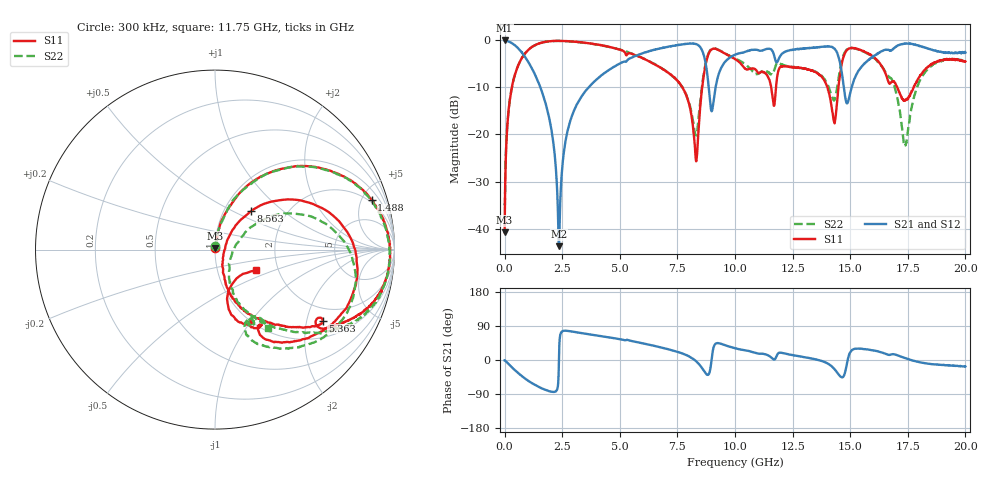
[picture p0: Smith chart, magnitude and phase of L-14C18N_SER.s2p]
!P/N: L-14C18NJV4
!Agilent N5230A: A.07.50.26
!Date: Tuesday, October 28, 2008 10:37:53
!Correction: S11(Full 2 Port(1,2))
!S21(Full 2 Port(1,2))
!S12(Full 2 Port(1,2))
!S22(Full 2 Port(1,2))
!S2P File: Measurements: S11, S21, S12, S22:
# Hz S  dB  R 50
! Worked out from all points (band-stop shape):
!   1601 points, 300 kHz to 20 GHz, reference 50 ohm
!   highest |S21| = -0.12 dB at 300 kHz (marker M1); lowest = -43.7 dB at 2.363 GHz (marker M2)
!   |S21| within 3 dB of the highest: 5.822 GHz to 8.64 GHz (2.817 GHz wide, 39 % of centre); 16.13 GHz to end of sweep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
!   lowest |S11| = -40.8 dB at 300 kHz (marker M3), VSWR 1.02, Z = 49.9 + j0.912 ohm
!   |S11| at or under -10 dB: 7.709 GHz to 8.575 GHz (865.7 MHz wide, 10.6 % of centre); 14 GHz to 14.49 GHz (487.4 MHz wide, 3.42 % of centre); 17.04 GHz to 17.76 GHz (714.2 MHz wide, 4.11 % of centre)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
!   |S22| runs from -34.9 to -0.2 dB; largest |S21 - S12| = 0.022
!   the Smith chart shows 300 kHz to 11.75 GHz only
!   S11 on the Smith chart (normalised r, x): 300 kHz: 1.00, +0.02; 1.488 GHz: 1.76, +5.98; 5.363 GHz: 1.53, -2.49; 8.563 GHz: 1.34, +0.63; 11.75 GHz: 1.54, -0.38
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300000  -40.76 94.4  -0.12 -0.9  -0.14 -0.5  -34.64 96.2
3.627946e8  -8.93 65.7  -0.85 -22.1  -0.85 -22.1  -8.96 65.5
1.487778e9  -0.77 17.5  -9.23 -71.4  -9.24 -71.4  -0.78 17.2
2.037769e9  -0.26 3.3  -19.18 -83.7  -19.20 -83.9  -0.27 2.4
2.362765e9  -0.20 -3.2  -43.66 14.0  -43.53 12.5  -0.22 -4.4
2.70026e9  -0.26 -8.4  -19.98 77.1  -20.00 77.1  -0.28 -10.2
3.33775e9  -0.52 -16.4  -12.00 70.8  -11.99 70.7  -0.55 -18.7
5.36272e9  -2.88 -33.4  -4.12 52.5  -4.13 52.6  -2.63 -38.9
6.6752e9  -5.62 -52.2  -1.88 34.7  -1.84 34.4  -5.61 -53.7
7.825183e9  -11.08 -70.1  -0.85 14.4  -0.88 14.5  -11.03 -67.2
8.300176e9  -25.37 -29.4  -0.88 -2.4  -0.87 -2.5  -20.16 -22.4
8.562672e9  -10.57 46.9  -2.10 -20.9  -2.12 -21.0  -9.96 31.6
9.000165e9  -1.98 -6.2  -15.03 9.2  -15.03 9.2  -1.88 -14.3
1.000015e10  -4.06 -55.3  -3.13 31.1  -3.16 31.0  -3.94 -59.4
1.175012e10  -11.77 -26.8  -4.26 3.3  -4.24 3.4  -5.61 -56.0
1.33376e10  -6.53 -76.7  -1.65 3.7  -1.73 3.8  -6.42 -88.1
1.431259e10  -17.35 -39.5  -1.82 -23.7  -1.86 -23.6  -12.59 -51.2
1.482508e10  -2.36 -15.8  -13.14 -19.5  -13.13 -20.0  -2.20 -38.8
1.667505e10  -9.08 -39.2  -2.14 13.5  -2.15 13.6  -7.85 -73.1
1.738754e10  -12.85 11.0  -0.80 5.0  -0.81 4.8  -22.23 -176.5
1.825003e10  -6.29 60.8  -1.66 -8.5  -1.60 -8.6  -6.84 91.7
2e10  -4.56 60.4  -2.67 -17.1  -2.64 -18.5  -4.51 82.4
